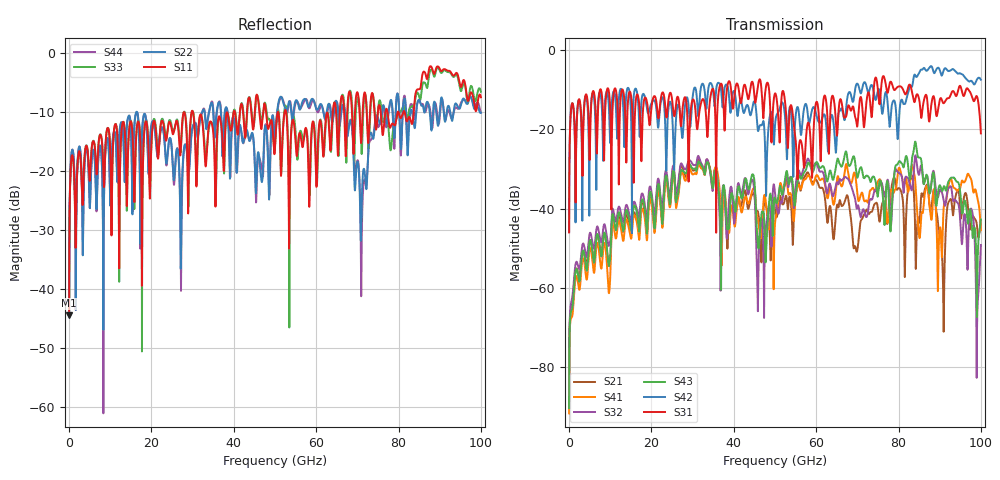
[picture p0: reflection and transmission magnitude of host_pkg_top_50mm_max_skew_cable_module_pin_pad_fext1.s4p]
# Hz S RI R 50
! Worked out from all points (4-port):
!   10000 points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, 10 MHz to 100 GHz, reference 50 ohm
!   strongest paths, dB at 10 MHz, 25.01 GHz, 50.01 GHz, 75.01 GHz, 100 GHz:
!     S31: -46.0, -12.4, -10.9, -10.2, -21.0
!     S42: -45.9, -16.0, -18.9, -10.1, -7.5
!     S43: -90.3, -32.7, -37.4, -36.6, -42.7
!     S32: -88.6, -30.8, -36.1, -35.6, -49.2
!     S41: -91.6, -33.7, -43.6, -33.1, -45.4
!     S21: -89.7, -31.7, -40.5, -40.1, -43.8
!   lowest |S11| = -44.4 dB at 10 MHz (marker M1), VSWR 1.01, Z = 50.3 + j0.533 ohm
!   |S11| at or under -10 dB: start of sweep to 27.87 GHz; 30.09 GHz to 39.95 GHz (9.868 GHz wide, 28.2 % of centre); 52.71 GHz to 64.04 GHz (11.34 GHz wide, 19.4 % of centre)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
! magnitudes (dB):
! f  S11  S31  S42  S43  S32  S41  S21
! 10 MHz  -44.4  -46.0  -45.9  -90.3  -88.6  -91.6  -89.7
! 5.85 GHz  -14.9  -10.3  -11.0  -52.4  -49.6  -55.0  -51.8
! 31.46 GHz  -12.3  -17.1  -15.8  -28.1  -26.8  -28.8  -27.4
! 45.85 GHz  -7.7  -9.0  -20.3  -49.0  -65.7  -42.6  -40.8
! 58.02 GHz  -17.3  -18.3  -16.7  -28.5  -27.4  -31.6  -30.9
! 71.05 GHz  -13.9  -12.8  -10.4  -29.9  -41.3  -36.0  -42.7
! 100 GHz  -7.5  -21.0  -7.5  -42.7  -49.2  -45.4  -43.8
